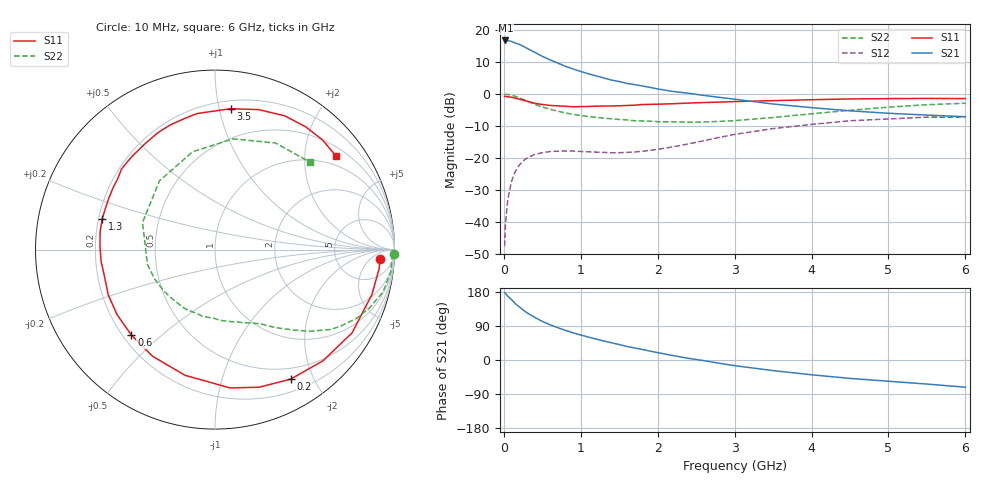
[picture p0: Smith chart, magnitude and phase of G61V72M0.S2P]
! SIEMENS Small Signal Semiconductors
! BFG193
! Si NPN RF Bipolar Junction Transistor in SOT223
! VCE = 1.75 V  IC = 2 mA
! Common Emitter S-Parameters:  August  1996
# GHz  S  MA  R  50
!  f  S11  S21  S12  S22
! GHz  MAG  ANG  MAG  ANG  MAG  ANG  MAG  ANG
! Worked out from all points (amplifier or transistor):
!   36 points, 10 MHz to 6 GHz, reference 50 ohm
!   highest |S21| = 16.8 dB at 20 MHz (marker M1)
!   |S21| within 3 dB of that: start of sweep to 345.3 MHz
!   unconditionally stable (mu >= 1): 1.357 GHz to 2.747 GHz
!   at 250 MHz: K = 0.18, MSG = 17.9 dB, |S12| = -20.9 dB
!   at 1.4 GHz: K = 1.04, MAG = 10.1 dB, |S12| = -18.4 dB
!   at 6 GHz: K = 0.98, MSG = 0.1 dB, |S12| = -7.2 dB
!   S11 on the Smith chart (normalised r, x): 10 MHz: 17, -11; 200 MHz: 0.35, -1.69; 600 MHz: 0.23, -0.40; 1.3 GHz: 0.21, +0.13; 3.5 GHz: 0.26, +1.08; 6 GHz: 0.72, +2.75
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0.01  0.9202 -3.2  6.874 177.7  0.0042 89.6  0.995 -1.5
0.02  0.9209 -6.5  6.898 176.5  0.009 91.4  0.9875 -2.8
0.05  0.9096 -15.9  6.852 168.5  0.022 81.0  0.9871 -7.2
0.1  0.8936 -31.3  6.653 159.6  0.0434 73.5  0.9655 -14.1
0.15  0.8635 -45.9  6.294 148.6  0.0623 64.2  0.9213 -20.5
0.2  0.8359 -59.7  5.999 140.5  0.0774 57.5  0.879 -25.7
0.25  0.8053 -72.2  5.612 132.0  0.0903 51.0  0.8263 -30.7
0.3  0.7753 -83.8  5.21 124.8  0.1004 45.9  0.7839 -34.6
0.4  0.7197 -103.5  4.516 112.8  0.1137 36.9  0.6963 -40.8
0.5  0.6884 -120.4  3.892 101.8  0.1216 29.9  0.6287 -45.5
0.6  0.6662 -134.3  3.436 93.1  0.1265 25.0  0.5802 -49.4
0.7  0.655 -146.4  3.058 85.3  0.1282 21.4  0.5417 -53.0
0.8  0.646 -157.1  2.728 78.2  0.1289 18.2  0.5077 -56.0
1.1  0.6411 178.3  2.077 60.4  0.1253 14.3  0.4463 -66.1
1.3  0.6512 165.0  1.789 50.2  0.1229 14.4  0.4202 -73.1
1.6  0.6644 148.7  1.469 35.7  0.123 17.5  0.3951 -86.0
2.2  0.7073 123.4  1.1 11.7  0.1501 25.7  0.3699 -116.7
2.8  0.7497 103.1  0.891 -8.6  0.2105 23.7  0.3743 -154.5
3.5  0.79 83.6  0.7 -28.0  0.2892 9.8  0.4311 159.5
4.5  0.8406 62.5  0.548 -48.6  0.3831 -13.4  0.559 102.9
5.5  0.8558 45.7  0.47 -63.5  0.4369 -40.5  0.6831 60.4
6  0.8519 37.8  0.443 -71.8  0.4374 -55.2  0.7192 42.7
